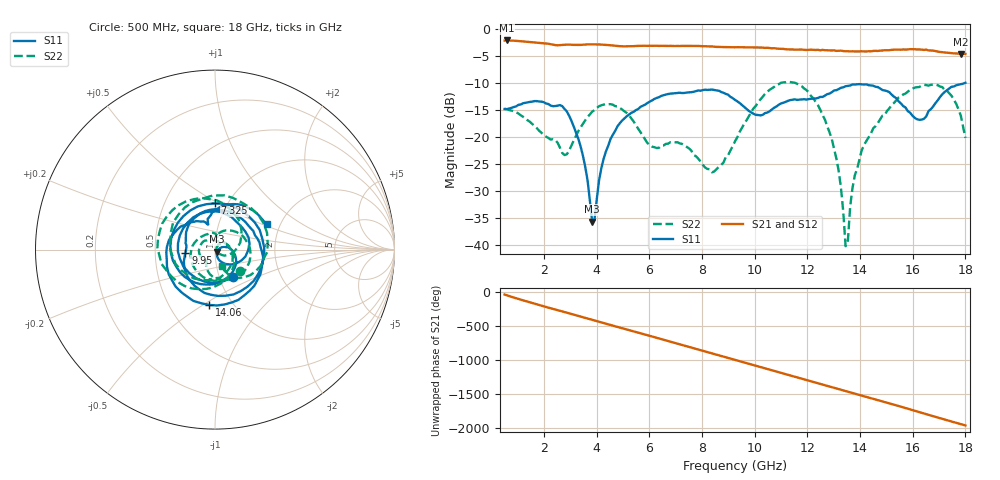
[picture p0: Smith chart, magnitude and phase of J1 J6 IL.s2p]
!Agilent Technologies,N5230A,MY45001360,A.07.50.67
!Agilent N5230A: A.07.50.67
!Date: Tuesday, April 16, 2024 16:32:21
!Correction: S11(Full 2 Port(1,2))
!S21(Full 2 Port(1,2))
!S12(Full 2 Port(1,2))
!S22(Full 2 Port(1,2))
!S2P File: Measurements: S11, S21, S12, S22:
# Hz S  dB  R 50
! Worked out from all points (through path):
!   201 points, 500 MHz to 18 GHz, reference 50 ohm
!   highest |S21| = -2.04 dB at 587.5 MHz (marker M1); lowest = -4.5 dB at 17.82 GHz (marker M2)
!   group delay of S21, straight-line fit = 303 ps
!   lowest |S11| = -35.6 dB at 3.825 GHz (marker M3), VSWR 1.03, Z = 51.1 - j1.24 ohm
!   |S11| at or under -10 dB: start of sweep to 17.94 GHz
!   |S22| runs from -40.2 to -9.7 dB; largest |S21 - S12| = 0.0094
!   S11 on the Smith chart (normalised r, x): 500 MHz: 1.16, -0.37; 7.325 GHz: 0.87, +0.48; 9.95 GHz: 0.72, -0.02; 14.06 GHz: 0.78, -0.53; 18 GHz: 1.70, +0.53
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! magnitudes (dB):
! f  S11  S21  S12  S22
! 500 MHz  -14.7  -2.1  -2.0  -14.7
! 587.5 MHz  -14.8  -2.0  -2.0  -14.8
! 2.688 GHz  -14.2  -2.9  -2.9  -22.9
! 3.475 GHz  -23.4  -2.8  -2.8  -17.5
! 3.825 GHz  -35.6  -2.7  -2.8  -15.2
! 4.525 GHz  -20.3  -2.9  -2.9  -13.8
! 6.362 GHz  -12.6  -3.0  -3.0  -21.9
! 7.325 GHz  -11.8  -3.1  -3.1  -21.5
! 8.375 GHz  -11.1  -3.1  -3.2  -26.5
! 9.25 GHz  -13.1  -3.3  -3.3  -20.7
! 9.95 GHz  -15.6  -3.3  -3.3  -14.6
! 11 GHz  -13.7  -3.6  -3.6  -9.9
! 12.22 GHz  -12.8  -3.8  -3.7  -12.7
! 13.1 GHz  -11.3  -4.0  -4.0  -23.9
! 13.45 GHz  -10.5  -4.0  -4.0  -40.2
! 13.71 GHz  -10.2  -4.0  -4.1  -29.4
! 14.06 GHz  -10.2  -4.0  -4.0  -22.4
! 15.11 GHz  -11.6  -3.8  -3.8  -14.6
! 16.34 GHz  -16.7  -3.7  -3.7  -10.4
! 17.12 GHz  -12.0  -4.2  -4.2  -10.7
! 17.82 GHz  -10.2  -4.5  -4.4  -16.0
! 18 GHz  -9.9  -4.5  -4.5  -20.1
